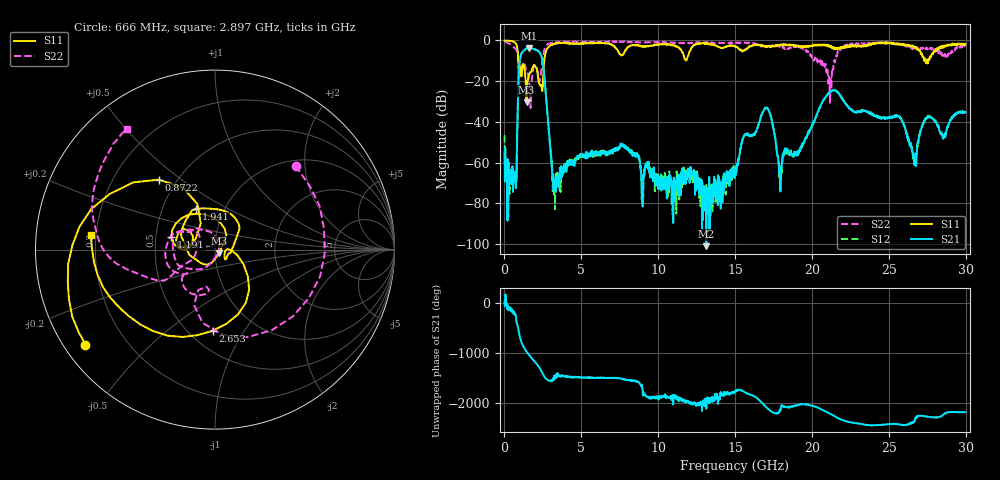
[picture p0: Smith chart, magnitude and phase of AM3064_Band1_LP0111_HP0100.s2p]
# Hz S DB R 50.0
!freq dBS11 angS11 dBS21 angS21 dBS12 angS12 dBS22 angS22
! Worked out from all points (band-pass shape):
!   1600 points, 10 MHz to 29.98 GHz, reference 50 ohm
!   highest |S21| = -3.72 dB at 1.584 GHz (marker M1); lowest = -101.1 dB at 13.13 GHz (marker M2)
!   |S21| within 3 dB of the highest: 1.091 GHz to 2.349 GHz (1.258 GHz wide, 73.1 % of centre)
!   lowest |S11| = -30.4 dB at 1.435 GHz (marker M3), VSWR 1.06, Z = 52.3 - j2.07 ohm
!   |S11| at or under -10 dB: 902.1 MHz to 2.587 GHz (1.685 GHz wide, 96.6 % of centre); 27.39174 GHz to 27.46025 GHz (68.51 MHz wide, 0.25 % of centre); 27.49002 GHz to 27.56432 GHz (74.3 MHz wide, 0.27 % of centre)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
!   |S22| runs from -33.2 to -0.3 dB; largest |S21 - S12| = 0.0088
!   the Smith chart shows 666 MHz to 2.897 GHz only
!   S11 on the Smith chart (normalised r, x): 666 MHz: 0.06, -0.33; 872.2 MHz: 0.40, +0.41; 1.191 GHz: 0.60, +0.09; 1.941 GHz: 0.74, +0.36; 2.653 GHz: 0.65, -0.73; 2.897 GHz: 0.18, +0.06
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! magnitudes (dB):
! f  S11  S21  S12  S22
! 10 MHz  -0.1  -55.1  -46.6  -0.3
! 666 MHz  -1.0  -64.8  -65.0  -3.8
! 872.2 MHz  -6.0  -30.6  -30.6  -7.7
! 1.191 GHz  -12.0  -5.5  -5.5  -11.5
! 1.435 GHz  -30.4  -4.0  -3.9  -15.6
! 1.584 GHz  -17.3  -3.7  -3.7  -19.0
! 1.941 GHz  -12.0  -4.4  -4.3  -12.8
! 2.653 GHz  -6.9  -22.7  -22.7  -3.4
! 2.897 GHz  -3.1  -45.3  -45.0  -1.6
! 3.29 GHz  -1.7  -71.1  -82.9  -0.9
! 5.015 GHz  -1.5  -56.6  -56.9  -0.7
! 10 GHz  -2.1  -66.8  -68.1  -0.9
! 13.13 GHz  -1.6  -101.1  -70.8  -1.0
! 15 GHz  -3.0  -63.5  -63.6  -1.4
! 16.97 GHz  -2.8  -33.3  -33.4  -2.9
! 17.93 GHz  -2.0  -65.6  -64.6  -2.6
! 19.99 GHz  -2.9  -42.0  -42.4  -8.2
! 21.38 GHz  -3.2  -24.6  -24.5  -14.6
! 25 GHz  -1.1  -37.9  -38.3  -1.2
! 26.68 GHz  -3.1  -59.7  -59.0  -4.1
! 27.45 GHz  -10.4  -38.2  -38.1  -3.6
! 29.98 GHz  -1.7  -35.3  -35.1  -2.9
